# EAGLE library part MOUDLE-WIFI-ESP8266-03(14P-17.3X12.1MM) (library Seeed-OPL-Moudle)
317060012
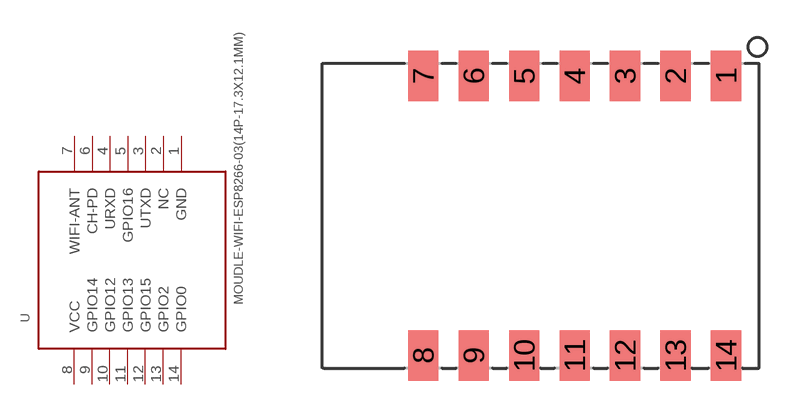
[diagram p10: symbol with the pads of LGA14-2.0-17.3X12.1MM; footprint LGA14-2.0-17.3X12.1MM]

Designator prefix U

## MOUDLE-WIFI-ESP8266-03(14P-17.3X12.1MM) (MPN: ESP8266-ESP-03; VALUE: ESP8266-ESP-03)  [LGA14-2.0-17.3X12.1MM]
1  GND
2  NC
3  UTXD
4  URXD
5  GPIO16
6  CH-PD
7  WIFI-ANT
8  VCC
9  GPIO14
10  GPIO12
11  GPIO13
12  GPIO15
13  GPIO2
14  GPIO0

## Footprint LGA14-2.0-17.3X12.1MM (pad centres in mm)
smd 1.2 x 2: 1 7.35,5.55; 2 5.35,5.55; 3 3.35,5.55; 4 1.35,5.55; 5 -0.65,5.55; 6 -2.65,5.55; 7 -4.65,5.55; 8 -4.65,-5.55; 9 -2.65,-5.55; 10 -0.65,-5.55; 11 1.35,-5.55; 12 3.35,-5.55; 13 5.35,-5.55; 14 7.35,-5.55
